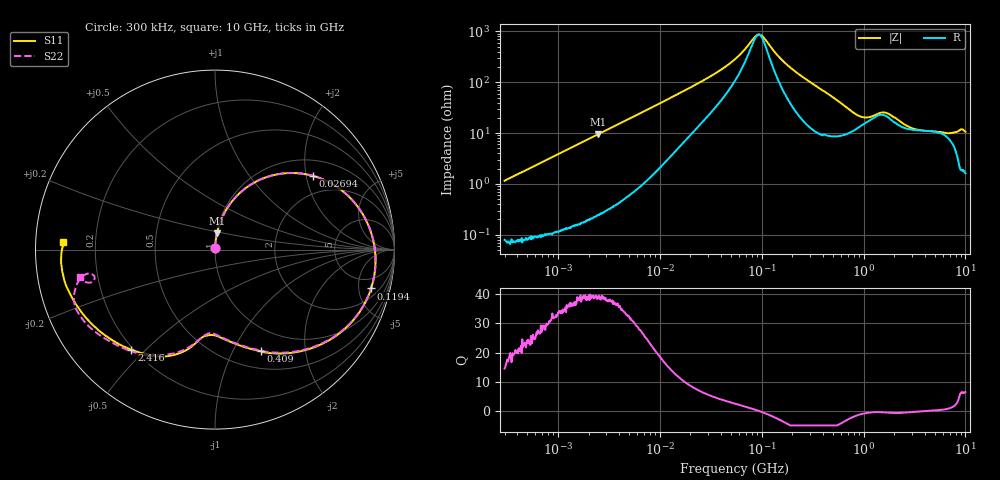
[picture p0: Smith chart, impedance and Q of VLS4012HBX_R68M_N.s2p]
! S-Parameter Data Generated by TDK Corporation
! Copyright(C) 2023 TDK Corporation.
! All Rights Reserved.
! TDK P/N: VLS4012HBX-R68M-N (Inductor)
! Property: L=680nH at 1MHz
! Size(LxWxT): 4x4x1.2mm
! Model Type: s2p (Touchstone File Format Version 1.0)
! Frequency: DC=Yes Start=0.3MHz Stop=10000MHz 802points Log-sweep
! Model Generated on June 16, 2023
! Port Assignments:
!  1 ---@@@--- 2
! Applicable Conditions:
!  Temperature = 25 degC
!  DC Bias Current = 0 A
!  Small Signal Operation
! Terms and conditions regarding TDK Simulation Models
! (1)This simulation model is being provided solely for informational purposes. Please refer to the specifications of the products in terms of detailed characteristics of such products.
! (2)In no event shall TDK Corporation of any of its subsidiaries be liable for any loss or damage arising, directly or indirectly,
!  From any information contained in this simulation model, including, but not limited to loss or damages arising from any inaccuracies, omissions or errors in connection with such information.
! (3)Any and all copyrights on this simulation model are owned by TDK Corporation.
!  Duplication or redistribution of this simulation model without prior written permission from TDK Corporation is prohibited.
! (4)This simulation model is subject to any modification or change without any prior notice.
! (5)Neither TDK Corporation nor any of its subsidiaries shall make any warranty, express or implied,
!  Including but not limited to the correctness, implied warranties of merchantability and fitness for a particular purpose with respect to this simulation models.
! (6)The use of this simulation model shall be deemed to have consented to the terms and conditions hereof.
# Hz S MA R 50
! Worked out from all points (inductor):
!   801 points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, 300 kHz to 10 GHz, reference 50 ohm
!   read as one part in series: L = 613 nH near 318.3 kHz
!   highest Q = 39.3 at 2.47 MHz (marker M1), where L = 606 nH
!   self-resonance near 93.33 MHz
!   S11 on the Smith chart (normalised r, x): 300 kHz: 1.00, +0.02; 26.94 MHz: 1.42, +2.19; 119.4 MHz: 3.09, -6.79; 409 MHz: 0.70, -1.29; 2.416 GHz: 0.19, -0.45; 10 GHz: 0.08, +0.03
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300000  0.0113 85.4  0.9989 -0.7  0.9993 -0.7  0.01117 85.2
1713600  0.06438 84.7  0.9961 -3.8  0.9963 -3.8  0.06444 84.7
2469661  0.09235 83.1  0.9931 -5.4  0.9935 -5.4  0.09235 83.1
9671944  0.3395 66.7  0.9229 -20.3  0.923 -20.3  0.3395 66.7
1.740512e7  0.5357 51.1  0.7923 -33.1  0.7924 -33.1  0.5357 51.2
2.693747e7  0.6827 37.0  0.6288 -43.7  0.6288 -43.7  0.6827 37.1
5.477226e7  0.8471 13.3  0.2997 -54.4  0.2998 -54.4  0.8472 13.5
9.209736e7  0.8968 -4.3  0.1033 -7.9  0.1034 -7.9  0.897 -4.1
1.014901e8  0.8989 -7.8  0.1101 17.2  0.1101 17.2  0.8991 -7.5
1.19394e8  0.8964 -14.0  0.166 41.7  0.1661 41.7  0.8966 -13.6
1.810762e8  0.8487 -31.1  0.3807 47.2  0.3807 47.2  0.8489 -30.6
3.126428e8  0.7033 -55.2  0.6368 28.9  0.6369 28.9  0.7032 -54.5
4.089972e8  0.6197 -65.8  0.7151 18.3  0.7151 18.2  0.6197 -65.2
7.956093e8  0.4817 -88.7  0.7809 -9.9  0.781 -10.0  0.476 -88.8
1.212691e9  0.4986 -98.8  0.7035 -28.5  0.7036 -28.5  0.4935 -98.5
1.767019e9  0.6417 -112.9  0.5863 -40.4  0.5864 -40.4  0.6372 -113.8
2.416286e9  0.7272 -129.9  0.5325 -51.0  0.5326 -51.0  0.7291 -128.4
5.21579e9  0.8378 -160.5  0.3243 -82.5  0.3243 -82.5  0.8325 -151.7
7.06055e9  0.8584 -170.6  0.2693 -95.3  0.2693 -95.3  0.8303 -161.2
8.322921e9  0.8572 -177.9  0.2354 -105.0  0.2354 -105.1  0.7369 -169.1
8.993752e9  0.8485 178.9  0.2188 -106.5  0.2189 -106.5  0.6892 -166.5
1e10  0.8457 177.1  0.2245 -109.7  0.2245 -109.8  0.7695 -168.5
